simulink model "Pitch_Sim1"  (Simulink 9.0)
settings: Solver=ode45  StartTime=0.0  StopTime=100  RelTol=1e-3  EnableMultiTasking=on
InitFcn:
  | init
StartFcn:
  | init
StopFcn:
  | pl
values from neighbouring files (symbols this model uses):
  d2r = 1/r2d    (= 0.0174532925199)    [freq.m]    (also in init.m; frequ.m; init_lat.m; pl.m)
undefined symbols (not defined in the file or in its folder): Ap, Bp, Cp, Dp

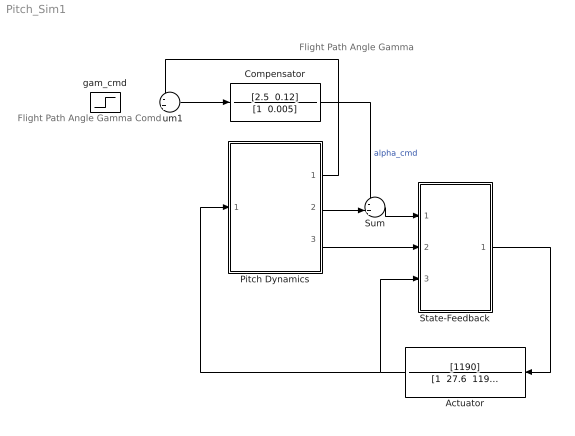
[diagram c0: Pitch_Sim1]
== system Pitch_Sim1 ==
  note: Flight Path Angle Gamma Comd
  note: Flight Path Angle Gamma
  Actuator : TransferFcn  Numerator=[1190]  Denominator="[1  27.6  1190]"
  Compensator : TransferFcn  Numerator="[2.5  0.12]"  Denominator="[1  0.005]"
  Pitch Dynamics : Subsystem
  State-Feedback : Subsystem
  Sum : Sum  Inputs=-+|
  Sum1 : Sum  Inputs=-+|
  gam_cmd : Step  Time=0  After=1*d2r  SampleTime=0
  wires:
  Sum/1 -> State-Feedback/1(alfa)
  Compensator/1 -> Sum/1  "alpha_cmd"
  Sum1/1 -> Compensator/1
  Pitch Dynamics/2(alpha_sens) -> Sum/2
  Pitch Dynamics/3(q) -> State-Feedback/2(q)
  State-Feedback/1(delv_cmd) -> Actuator/1
  Actuator/1 -> Pitch Dynamics/1(Elev), State-Feedback/3(d-elev)
  Pitch Dynamics/1(gamma) -> Sum1/1

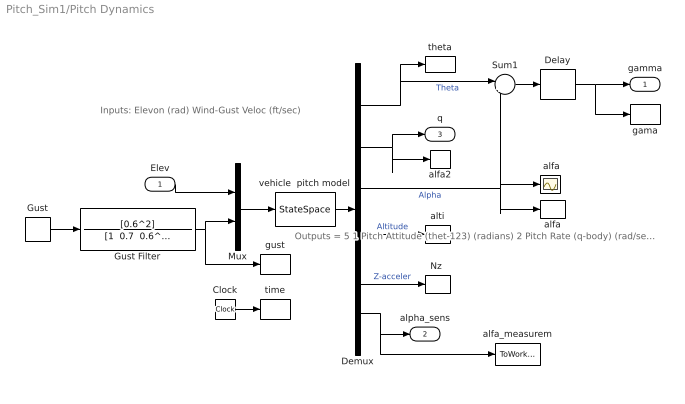
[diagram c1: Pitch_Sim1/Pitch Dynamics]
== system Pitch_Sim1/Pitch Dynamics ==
  note: Inputs: Elevon (rad) Wind-Gust Veloc (ft/sec)
  note: Outputs = 5 1 Pitch Attitude (thet-123) (radians) 2 Pitch Rate (q-body) (rad/sec) 3 Angle of attack, alfa, (radians) 4 Change in Altitude, delta-H, (feet) 5 Z-Acceleromet, (ft/sec^2) Translation 6 Alpha Sensed at Vane (radian)
  Elev : Inport
  " alfa" : Scope
  Clock : Clock
  Delay : TransportDelay  PadeOrder=2
  Demux : Demux  Outputs=6
  Gust : DiscretePulseGenerator  PulseType=Time based  Amplitude=30  Period=500  PulseWidth=2  PhaseDelay=10
  Gust Filter : TransferFcn  Numerator=[0.6^2]  Denominator="[1  0.7  0.6^2]"
  Mux : Mux  Inputs=2
  "Nz " : ToWorkspace  VariableName=Nz  SampleTime=-1
  Sum1 : Sum  Inputs=|+-
  alfa : ToWorkspace  VariableName=alfa  SampleTime=-1
  alfa2 : ToWorkspace  VariableName=q  SampleTime=-1
  alfa_measurem : ToWorkspace  VariableName=alfa_est  SampleTime=-1
  alti : ToWorkspace  VariableName=dH  SampleTime=-1
  gama : ToWorkspace  VariableName=gama  SampleTime=-1
  gust : ToWorkspace  VariableName=Vgst  SampleTime=-1
  theta : ToWorkspace  VariableName=theta  SampleTime=-1
  time : ToWorkspace  VariableName=time  SampleTime=-1
  vehicle  pitch model : StateSpace  A=Ap  B=Bp  C=Cp  D=Dp  InitialCondition=0
  gamma : Outport
  alpha_sens : Outport  Port=2
  q : Outport  Port=3
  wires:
  Mux/1 -> vehicle  pitch model/1
  Demux/1 -> Sum1/1, theta/1  "Theta"
  Demux/2 -> alfa2/1, q/1
  Elev/1 -> Mux/1
  Demux/3 -> " alfa"/1, alfa/1, Sum1/2  "Alpha"
  Gust Filter/1 -> Mux/2, gust/1
  Demux/5 -> "Nz "/1  "Z-acceler"
  Demux/6 -> alfa_measurem/1, alpha_sens/1
  Sum1/1 -> Delay/1
  Clock/1 -> time/1
  Gust/1 -> Gust Filter/1
  vehicle  pitch model/1 -> Demux/1
  Demux/4 -> alti/1  "Altitude"
  Delay/1 -> gamma/1, gama/1

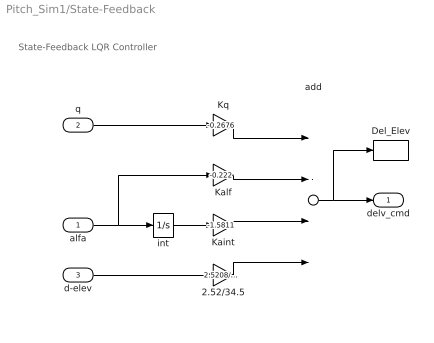
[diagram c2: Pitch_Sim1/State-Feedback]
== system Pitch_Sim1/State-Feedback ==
  note: State-Feedback LQR Controller
  alfa : Inport
  q : Inport  Port=2
  d-elev : Inport  Port=3
  2.52/34.5 : Gain  Gain=2.5208/34.5
  Del_Elev : ToWorkspace  VariableName=delev  SampleTime=-1
  Kaint : Gain  Gain=-1.5811
  Kalf : Gain  Gain=-0.222
  Kq : Gain  Gain=-0.2676
  add : Sum  Inputs=----
  int : Integrator
  delv_cmd : Outport
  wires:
  alfa/1 -> int/1, Kalf/1
  int/1 -> Kaint/1
  Kq/1 -> add/1
  Kalf/1 -> add/2
  Kaint/1 -> add/3
  2.52/34.5/1 -> add/4
  d-elev/1 -> 2.52/34.5/1
  q/1 -> Kq/1
  add/1 -> delv_cmd/1, Del_Elev/1
